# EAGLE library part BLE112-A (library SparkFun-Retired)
BlueGiga Bluetooth 4.0 module Bluetooth 4.0 module with integrated chip antenna and onboard 8051 processor and peripherals.
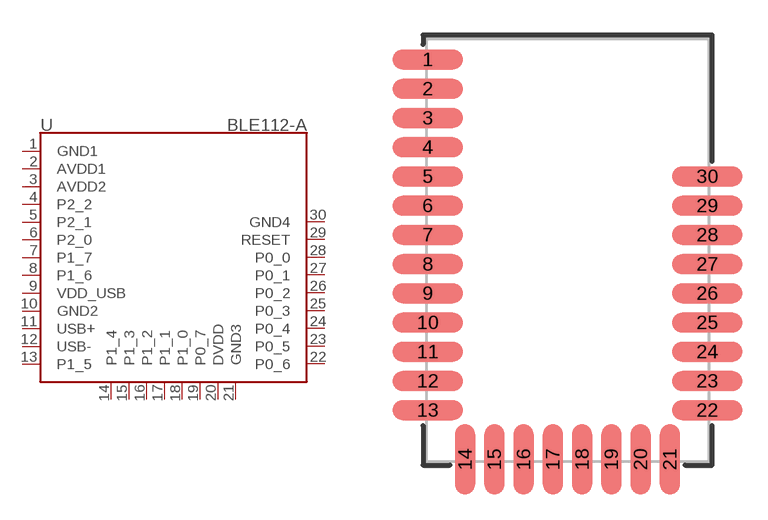
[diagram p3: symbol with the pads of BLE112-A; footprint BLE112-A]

Designator prefix U

## BLE112-A  [BLE112-A]
1  GND1
2  AVDD1
3  AVDD2
4  P2_2
5  P2_1
6  P2_0
7  P1_7
8  P1_6
9  VDD_USB
10  GND2
11  USB+
12  USB-
13  P1_5
14  P1_4
15  P1_3
16  P1_2
17  P1_1
18  P1_0
19  P0_7
20  DVDD
21  GND3
22  P0_6
23  P0_5
24  P0_4
25  P0_3
26  P0_2
27  P0_1
28  P0_0
29  RESET
30  GND4

## Footprint BLE112-A (pad centres in mm)
BLE112-A Bluetooth Smart Module Bluetooth 4.0 module with built-in chip antenna. Datasheet
smd 3 x 0.85: 1 -5.975,8.15; 2 -5.975,6.9; 3 -5.975,5.65; 4 -5.975,4.4; 5 -5.975,3.15; 6 -5.975,1.9; 7 -5.975,0.65; 8 -5.975,-0.6; 9 -5.975,-1.85; 10 -5.975,-3.1; 11 -5.975,-4.35; 12 -5.975,-5.6; 13 -5.975,-6.85; 22 5.975,-6.85; 23 5.975,-5.6; 24 5.975,-4.35; 25 5.975,-3.1; 26 5.975,-1.85; 27 5.975,-0.6; 28 5.975,0.65; 29 5.975,1.9; 30 5.975,3.15
smd 0.85 x 3: 14 -4.375,-8.95; 15 -3.125,-8.95; 16 -1.875,-8.95; 17 -0.625,-8.95; 18 0.625,-8.95; 19 1.875,-8.95; 20 3.125,-8.95; 21 4.375,-8.95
